FUNCTION_BLOCK FB_GetPtpDiag
VAR_IN_OUT
	arrNetId		: T_AmsNetIdArr;
	nSlaveAddr		: UINT;
END_VAR

VAR_INPUT
	bStart:BOOL;
END_VAR

VAR_OUTPUT
	bBusy:BOOL;
	bErr:BOOL;
	Errornumber:DWORD;
	Diag:		TPTP_DIAG;
END_VAR

VAR
	Flanke:			R_TRIG;
	fbRead:			FB_EcCoESdoReadEx;
	iState:			INT;
END_VAR

Flanke(CLK:=bStart);

IF Flanke.Q THEN
	bBusy:=TRUE;
	iState:=10;
END_IF

CASE iState OF
0:	bBusy:=FALSE;

10:	fbRead(sNetId:=F_CreateAmsNetId(arrNetId), nSlaveAddr:=nSlaveAddr);
	IF NOT fbRead.bBusy THEN
		fbRead.nSubIndex			:= 1;
		fbRead.nIndex				:= 16#FA80;
		fbRead.pDstBuf				:= ADR(Diag);
		fbRead.cbBufLen				:= SIZEOF(TPTP_DIAG);
		fbRead.bCompleteAccess		:= TRUE;
		fbRead.bExecute				:= TRUE;
		iState:=11;
	END_IF

11:	fbRead(sNetId:=F_CreateAmsNetId(arrNetId), nSlaveAddr:=nSlaveAddr);
	IF NOT fbRead.bBusy THEN
		IF NOT fbRead.bError THEN
			iState:=90;
		ELSE
			Errornumber				:= fbRead.nErrId;
			iState:=100;
		END_IF
		fbRead.bExecute				:= FALSE;
	END_IF

90:	(*Quit*)
	bErr:=FALSE;
	bStart:=FALSE;
	bBusy:=FALSE;
	iState:=0;

100:	(*Error*)
	bErr:=TRUE;
	bStart:=FALSE;
	bBusy:=FALSE;
	iState:=0;

END_CASE

END_FUNCTION_BLOCK
